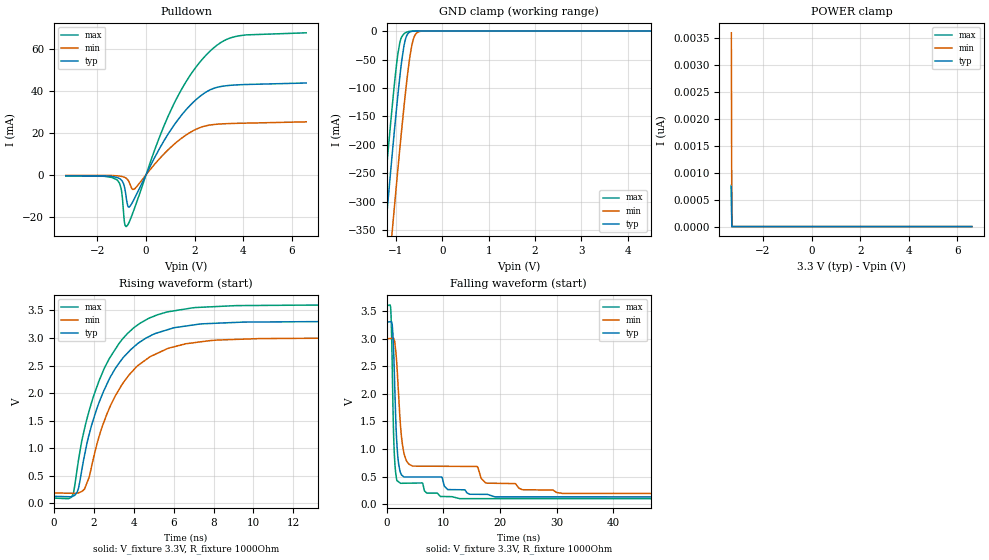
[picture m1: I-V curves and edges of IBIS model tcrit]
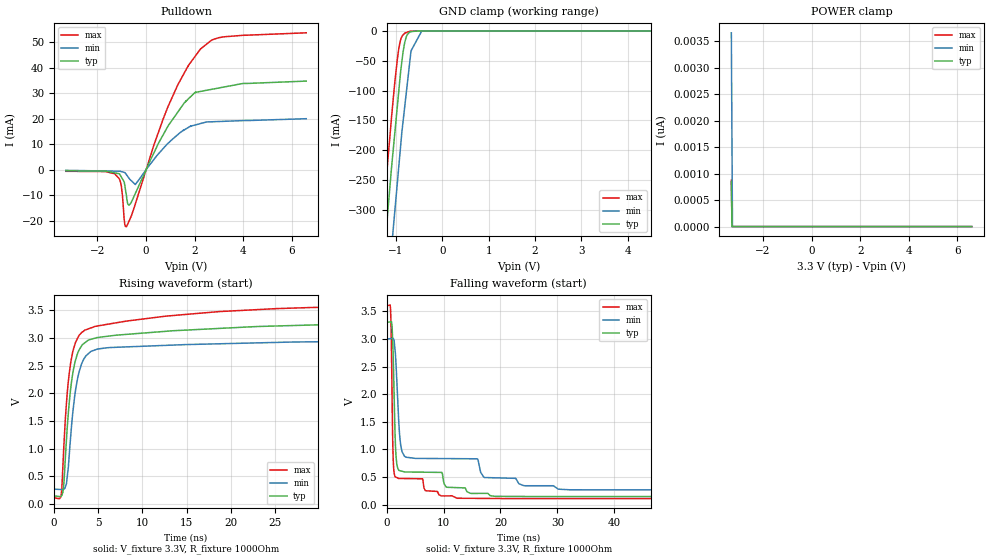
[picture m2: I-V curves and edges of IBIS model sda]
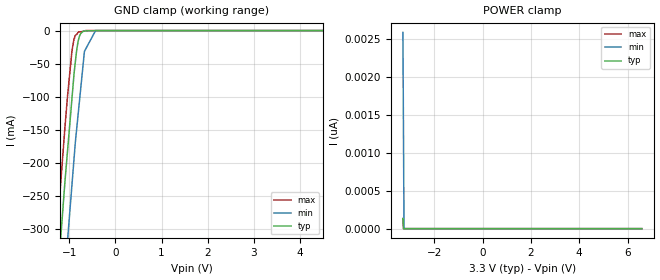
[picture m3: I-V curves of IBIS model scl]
| Texas Instruments Incorporated
| Quad Remote Diode and Local Temperature Sensor with SMBus Interface
| Marketing part#   Voltage Range   Package-type   #pins/pkg drawing
| LM95214NHL   3.0V - 3.6V   WSON   14-pin
[IBIS Ver]   4.1
[File name]   lm95214.ibs
[File Rev]   1.0
[Date]   07/07/2017
[Source]   Model built from spectre simulations at:
   Texas Instruments Incorporated.
   12500 TI Blvd
   Dallas, TX -75243
   For Support e-mail: odt-pfmodeling@list.ti.com
[Notes]   Revision History
   Rev 1.0: 07/07/2017
   - ccomp values are based on PVT settings:
   MIN: Low Voltage, High Temperature, Weak Process
   TYP: Nominal Voltage, Nominal Temperature, Nominal Process
   MAX: High Voltage, Low Temperature, Fast Process
   - C_comp although listed in numerical order of value are obtained from varying PVT conditions.
   For PVT conditions for each specific value, refer to the buffer description under respective [Model].
   IBIS model user is responsible for using appropriate C_comp to simulate for Signal Integrity.
[Disclaimer]  This model is designed as an aid for customers of Texas Instruments
 TI and its licensors and suppliers make no warranties, either expressed
 or implied, with respect to this  model, including the warranties of
 merchantability or fitness for a particular purpose.
 The model is provided solely on an "as is" basis. The entire risk as to
 its quality and performance is with the customer.
[Copyright] (C)Copyright 2017 Texas Instruments Incorporated.
   All rights reserved.
[Component]   LM95214NHL
[Manufacturer]  Texas Instruments Incorporated
[Package]   |14-pin WSON package
|   typ   min   max
R_pkg   0.005   0.005   0.005
L_pkg   0.20nH   0.2nH   0.2nH
C_pkg   0.6pF   0.6pF   0.6pF
[Pin]   signal_name   model_name   R_pin   L_pin   C_pin
1   NC   NC   0.005   0.2nH   0.6pF
2   VDD   POWER   0.005   0.2nH   0.6pF
3   D4+   NC   0.005   0.2nH   0.6pF
4   D3+   NC   0.005   0.2nH   0.6pF
5   D-   NC   0.005   0.2nH   0.6pF
6   D2+   NC   0.005   0.2nH   0.6pF
7   D1+   NC   0.005   0.2nH   0.6pF
8   GND   GND   0.005   0.2nH   0.6pF
9   A0   a0   0.005   0.2nH   0.6pF
10   TCRIT1B   tcrit   0.005   0.2nH   0.6pF
11   TCRIT2B   tcrit   0.005   0.2nH   0.6pF
12   SMBDAT   sda   0.005   0.2nH   0.6pF
13   SMBCLK   scl   0.005   0.2nH   0.6pF
14   TCRIT3B   tcrit   0.005   0.2nH   0.6pF
| Models and submodels in the file (4): tcrit (I/O_open_drain), sda (I/O_open_drain), scl (Input), a0 (Input)
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[Model]   tcrit
Model_type   I/O_open_drain
Polarity   Non-Inverting
Enable   Active-Low
Vmeas = 1.65
Vref = 3.3
Cref = 15pF
Rref = 50
Vinl = 0.33
Vinh = 2.97
|   typ   min   max
|   (nom PVT)   (fast PVT)   (slow PVT)
C_comp   0.674p   0.641p   0.723p
|C_comp (ON state)   0.674p   0.641p   0.723p
|C_comp (OFF state)   0.784p   0.758p   0.817p
[Model spec]
|subparameter
Vinl   0.33   0.3   0.36
Vinh   2.97   2.70   3.24
[Voltage Range]   3.3   3   3.6
[Temperature Range]   27   125   -40
[Pullup Reference]   3.3   3   3.6
[Pulldown Reference]   0   0   -0
[Power Clamp Reference]   3.3   3   3.6
[GND Clamp Reference]   0   0   0
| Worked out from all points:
|   slope of the pulldown table from 0 to 0.495 V, typ, clamps not added: 44 ohm
|   GND clamp passes 1 mA (typ) near -0.67 V on its own axis
|   falling waveform, V_fixture 3.3V, R_fixture 1000Ohm: 20-80 % time 805ps typ, 1.86ns min, 506ps max; typ from 3.3 V to 0.13 V
|   rising waveform, V_fixture 3.3V, R_fixture 1000Ohm: 20-80 % time 2.05ns typ, 2.1ns min, 2.02ns max; typ from 0.13 V to 3.3 V
[Pulldown]
|   Voltage   I(typ)   I(min)   I(max)
-3.3V     -506.6uA   -272.7uA   -674.3uA
-1.201V   -1.271mA   -495.5uA   -2.392mA
-1.023V   -2.435mA   -753.3uA   -6.801mA
-884.4mV  -5.998mA   -1.207mA   -22.99mA
-815.1mV  -10.88mA   -1.663mA   -24.7mA
-716.1mV  -15.46mA   -3.045mA   -23.14mA
-488.4mV  -11.54mA   -6.887mA   -16.42mA
976.8mV   20.67mA    12.68mA    29.68mA
1.67V     31.33mA    19.16mA    44.87mA
2.363V    38.68mA    23.06mA    55.77mA
3.61V     42.81mA    24.51mA    65.79mA
6.59V     43.8mA     25.26mA    67.75mA
[GND Clamp]
|   Voltage   I(typ)   I(min)   I(max)
-3.3V     -2.348A    -2.467A    -2.274A
-1.32V    -438.4mA   -575.6mA   -351.8mA
-1.27V    -391.9mA   -529.1mA   -305.4mA
-1.201V   -327.5mA   -464.5mA   -241.3mA
-1.112V   -246.2mA   -382.3mA   -161.3mA
-1.053V   -193.5mA   -328.3mA   -110.7mA
-914.1mV  -80.14mA   -206.3mA   -20.32mA
-825mV    -25.93mA   -133.1mA   -4.834mA
-765.6mV  -8.032mA   -88.59mA   -1.943mA
-636.9mV  -408.2uA   -18.8mA    -99.26uA
-488.4mV  -8.204uA   -748.6uA   -688.6nA
6.59V     0A         0A         0A
[POWER Clamp]
|   Voltage   I(typ)   I(min)   I(max)
-3.3V     743.6pA    3.593nA    765.9pA
-3.28V    0A         0A         0A
-3.27V    0A         0A         0A
6.59V     0A         0A         0A
[Ramp]
R_load = 1000
|   typ   min   max
dV/dt_r   1.9022/2.04818e-09   1.68542/2.08996e-09   2.10121/2.02466e-09
dV/dt_f   1.90221/8.05107e-10   1.68544/1.83982e-09   2.10122/5.0415e-10
[Falling Waveform]
V_fixture = 3.3V
V_fixture_min = 3V
V_fixture_max = 3.6V
R_fixture = 1000Ohm
C_fixture = 0F
|   Time   V(typ)   V(min)   V(max)
0s        3.3V       3V         3.6V
749.8ps   3.311V     3.007V     3.515V
992ps     3.262V     3.009V     2.533V
1.246ns   2.775V     3.009V     1.233V
1.751ns   1.212V     2.616V     460mV
2.562ns   545.2mV    1.294V     377.4mV
3.244ns   491.7mV    856.4mV    378.6mV
7.036ns   491.5mV    687.7mV    203.8mV
31.02ns   130.9mV    193.8mV    98.18mV
99.9ns    129.7mV    190.9mV    97.97mV
[Rising Waveform]
V_fixture = 3.3V
V_fixture_min = 3V
V_fixture_max = 3.6V
R_fixture = 1000Ohm
C_fixture = 0F
|   Time   V(typ)   V(min)   V(max)
0s        129.6mV    190.9mV    97.97mV
960ps     132.7mV    184.7mV    164mV
1.236ns   278.2mV    192mV      789.9mV
1.54ns    877.4mV    263.1mV    1.359V
1.779ns   1.267V     486.3mV    1.694V
2.272ns   1.838V     1.221V     2.23V
3.26ns    2.54V      2.062V     2.898V
4.819ns   3.037V     2.661V     3.367V
6.982ns   3.236V     2.913V     3.549V
99.9ns    3.3V       3V         3.6V
[Model]   sda
Model_type   I/O_open_drain
Polarity   Non-Inverting
Enable   Active-Low
Vmeas = 1.65
Vref = 3.3
Cref = 15pF
Rref = 50
Vinl = 0.33
Vinh = 2.97
|   typ   min   max
|   (nom PVT)   (fast PVT)   (slow PVT)
C_comp   0.674p   0.611p   0.730p
|C_comp (ON state)   0.674p   0.676p   0.730p
|C_comp (OFF state)   0.727p   0.676p   0.779p
[Model spec]
|subparameter
Vinl   0.33   0.3   0.36
Vinh   2.97   2.70   3.24
[Voltage Range]   3.3   3   3.6
[Temperature Range]   27   125   -40
[Pullup Reference]   3.3   3   3.6
[Pulldown Reference]   -0   -0   -0
[Power Clamp Reference]   3.3   3   3.6
[GND Clamp Reference]   0   0   0
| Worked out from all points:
|   slope of the pulldown table from 0 to 0.495 V, typ, clamps not added: 49 ohm
|   GND clamp passes 1 mA (typ) near -0.66 V on its own axis
|   falling waveform, V_fixture 3.3V, R_fixture 1000Ohm: 20-80 % time 584ps typ, 14.3ns min, 329ps max; typ from 3.3 V to 0.145 V
|   rising waveform, V_fixture 3.3V, R_fixture 1000Ohm: 20-80 % time 1.3ns typ, 1.27ns min, 1.35ns max; typ from 0.145 V to 3.3 V
[Pulldown]
|   Voltage   I(typ)   I(min)   I(max)
-3.3V     -439.9uA   -224.7uA   -597.8uA
-1.29V    -1.21mA    -543.3uA   -1.572mA
-1.042V   -2.437mA   -649.3uA   -5.14mA
-887.5mV  -5.38mA    -1.055mA   -20.49mA
-800.8mV  -10.69mA   -2.015mA   -22.27mA
-698.7mV  -13.83mA   -3.346mA   -20.09mA
-442.5mV  -9.316mA   -5.777mA   -13.44mA
914.4mV   17.31mA    10.45mA    25mA
1.636V    26.88mA    16mA       39.06mA
2.239V    30.71mA    18.11mA    47.32mA
3.181V    32.39mA    18.99mA    52.1mA
6.59V     34.76mA    20.02mA    53.68mA
[GND Clamp]
|   Voltage   I(typ)   I(min)   I(max)
-3.3V     -2.348A    -2.467A    -2.274A
-1.293V   -412.7mA   -550.1mA   -326.2mA
-1.267V   -389.2mA   -526mA     -302.9mA
-1.095V   -230.6mA   -366.8mA   -146.2mA
-1.069V   -209.6mA   -343.3mA   -124.7mA
-1.042V   -187.4mA   -319.6mA   -102mA
-930.8mV  -95.74mA   -222.3mA   -26.93mA
-847.2mV  -36.61mA   -153.6mA   -6.588mA
-800.8mV  -16.84mA   -121.6mA   -3.293mA
-673.2mV  -1.152mA   -33.36mA   -269uA
-442.5mV  0A         0A         -3.019uA
6.59V     0A         0A         0A
[POWER Clamp]
|   Voltage   I(typ)   I(min)   I(max)
-3.3V     849.1pA    3.66nA     876.3pA
-3.273V   0A         1.545nA    0A
-3.254V   0A         0A         0A
6.59V     0A         0A         0A
[Ramp]
R_load = 1000
|   typ   min   max
dV/dt_r   1.89284/1.28635e-09   1.64095/1.26054e-09   2.09437/1.34502e-09
dV/dt_f   1.89284/5.84033e-10   1.64095/1.41723e-08   2.09437/3.28744e-10
[Falling Waveform]
V_fixture = 3.3V
V_fixture_min = 3V
V_fixture_max = 3.6V
R_fixture = 1000Ohm
C_fixture = 0F
|   Time   V(typ)   V(min)   V(max)
0s        3.3V       3V         3.6V
700ps     3.311V     3.008V     3.541V
1.12ns    2.829V     3.013V     966.8mV
1.425ns   1.528V     2.867V     525.8mV
1.768ns   761.6mV    2.313V     493.7mV
2.24ns    618.7mV    1.335V     475.5mV
2.717ns   606.2mV    960.2mV    474.9mV
9.596ns   585.2mV    835.9mV    161mV
32.16ns   148.4mV    270.6mV    111.5mV
199.9ns   145.3mV    265.1mV    109.4mV
[Rising Waveform]
V_fixture = 3.3V
V_fixture_min = 3V
V_fixture_max = 3.6V
R_fixture = 1000Ohm
C_fixture = 0F
|   Time   V(typ)   V(min)   V(max)
0s        145.3mV    265.1mV    109.4mV
839.5ps   141.5mV    259.9mV    166.4mV
1.15ns    402.6mV    267.9mV    1.095V
1.425ns   1.158V     363.2mV    1.818V
1.994ns   2.203V     1.399V     2.631V
2.762ns   2.754V     2.327V     3.025V
4.266ns   2.981V     2.765V     3.188V
12.39ns   3.119V     2.867V     3.392V
45.1ns    3.279V     2.96V      3.589V
199.9ns   3.3V       3V         3.6V
[Model]   scl
Model_type   Input
Vinl = 0.33
Vinh = 2.97
|   typ   min   max
|   (nom PVT)   (fast PVT)   (slow PVT)
C_comp   0.364p   0.333p   0.397p
[Model spec]
|subparameter
Vinl   0.33   0.3   0.36
Vinh   2.97   2.70   3.24
[Voltage Range]   3.3   3   3.6
[Temperature Range]   27   125   -40
[Power Clamp Reference]   3.3   3   3.6
[GND Clamp Reference]   0   0   0
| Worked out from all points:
|   GND clamp passes 1 mA (typ) near -0.70 V on its own axis
[GND Clamp]
|   Voltage   I(typ)   I(min)   I(max)
-3.3V     -2.345A    -2.466A    -2.274A
-1.267V   -385.8mA   -525.4mA   -302.1mA
-1.095V   -227mA     -366mA     -144.9mA
-1.042V   -183.6mA   -318.8mA   -100.6mA
-943.1mV  -102mA     -232mA     -30.27mA
-912.1mV  -76.43mA   -204.9mA   -17.59mA
-847.2mV  -32.77mA   -152.4mA   -6.012mA
-800.3mV  -13.6mA    -119.7mA   -2.045mA
-748.2mV  -4.011mA   -83.51mA   -1.729mA
-673.2mV  -796.1uA   -31.35mA   -533.2uA
-431.7mV  -10.93uA   0A         0A
6.59V     0A         0A         0A
[POWER Clamp]
|   Voltage   I(typ)   I(min)   I(max)
-3.3V     134.5pA    2.588nA    131.1pA
-3.274V   0A         1.098nA    489.1fA
-3.254V   0A         0A         0A
6.59V     0A         0A         0A
